TYPE ST_AxisStatus :
STRUCT
	Current_Pos:LREAL;(*轴当前位置*)

	Axis_Ready:BOOL;(*NC轴准备好*)
	Axis_Err:BOOL;(*NC轴故障*)
	Axis_ErrID:UDINT;(*NC轴故障代码*)
	Axis_IsCalibrated:BOOL;(*NC轴寻参完成*)
	Axis_IsNotMoving:BOOL;(*NC轴静止*)
	Axis_IsPTP	:BOOL;
END_STRUCT
END_TYPE
